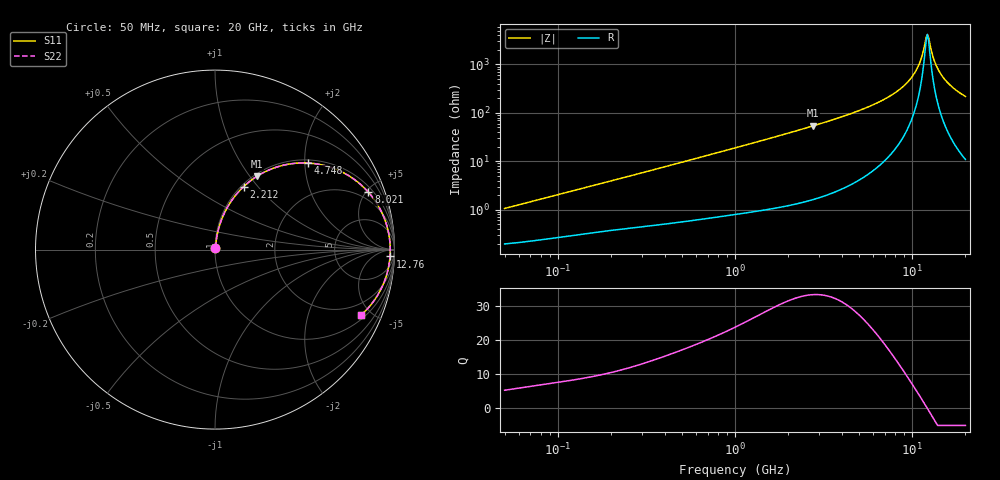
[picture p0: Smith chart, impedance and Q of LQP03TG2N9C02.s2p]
!Murata Part Number: LQP03TG2N9C02
!These Parameters are Measured in Series Mode Connection
!  o--[Z]--o
!Port1  Port2
!  o-------o
!Freq. Start=50[MHz] Stop=20[GHz], 401[Steps]
# Hz S RI R 50
!Freq.(Hz) S11(Real) S11(Imag) S21(Real) S21(Imag) S12(Real) S12(Imag) S22(Real) S22(Imag)
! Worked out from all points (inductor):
!   401 points, 50 MHz to 20 GHz, reference 50 ohm
!   read as one part in series: L = 3.29 nH near 51.52 MHz
!   highest Q = 33.3 at 2.769 GHz (marker M1), where L = 3.1 nH
!   self-resonance near 12.02 GHz
!   S11 on the Smith chart (normalised r, x): 50 MHz: 1.00, +0.02; 2.212 GHz: 1.03, +0.85; 4.748 GHz: 1.07, +2.06; 8.021 GHz: 1.36, +5.19; 12.76 GHz: 23, -37; 20 GHz: 1.22, -4.36
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5e7  0.00207 0.0104  0.9979 -0.0104  0.9979 -0.0104  0.00207 0.0104
1.364002e8  0.00384 0.027  0.9962 -0.027  0.9962 -0.027  0.00384 0.027
3.721004e8  0.00983 0.0703  0.9902 -0.0703  0.9902 -0.0703  0.00983 0.0703
1e9  0.0413 0.1791  0.9587 -0.1791  0.9587 -0.1791  0.0413 0.1791
2.211938e9  0.1597 0.3512  0.8403 -0.3512  0.8403 -0.3512  0.1597 0.3512
2.728004e9  0.2268 0.404  0.7732 -0.404  0.7732 -0.404  0.2268 0.404
2.769174e9  0.2324 0.4076  0.7676 -0.4076  0.7676 -0.4076  0.2324 0.4076
4.748272e9  0.5154 0.4825  0.4846 -0.4825  0.4846 -0.4825  0.5154 0.4825
5.944466e9  0.6671 0.4503  0.3329 -0.4503  0.3329 -0.4503  0.6671 0.4503
7.442007e9  0.8125 0.3618  0.1875 -0.3618  0.1875 -0.3618  0.8125 0.3618
8.020766e9  0.8548 0.3196  0.1452 -0.3196  0.1452 -0.3196  0.8548 0.3196
9.316812e9  0.9236 0.2184  0.0764 -0.2184  0.0764 -0.2184  0.9236 0.2184
1.034674e10  0.9562 0.1372  0.0438 -0.1372  0.0438 -0.1372  0.9562 0.1372
1.115139e10  0.9703 0.0757  0.0297 -0.0757  0.0297 -0.0757  0.9703 0.0757
1.201863e10  0.9763 0.0126  0.0237 -0.0126  0.0237 -0.0126  0.9763 0.0126
1.220001e10  0.9765 -5.99e-05  0.0235 5.99e-05  0.0235 5.99e-05  0.9765 -5.99e-05
1.238412e10  0.9764 -0.0128  0.0236 0.0128  0.0236 0.0128  0.9764 -0.0128
1.276073e10  0.9752 -0.0381  0.0248 0.0381  0.0248 0.0381  0.9752 -0.0381
1.354865e10  0.9688 -0.0884  0.0312 0.0884  0.0312 0.0884  0.9688 -0.0884
1.482269e10  0.9495 -0.1617  0.0505 0.1617  0.0505 0.1617  0.9495 -0.1617
1.696185e10  0.9008 -0.2627  0.0992 0.2627  0.0992 0.2627  0.9008 -0.2627
2e10  0.8146 -0.3644  0.1854 0.3644  0.1854 0.3644  0.8146 -0.3644
